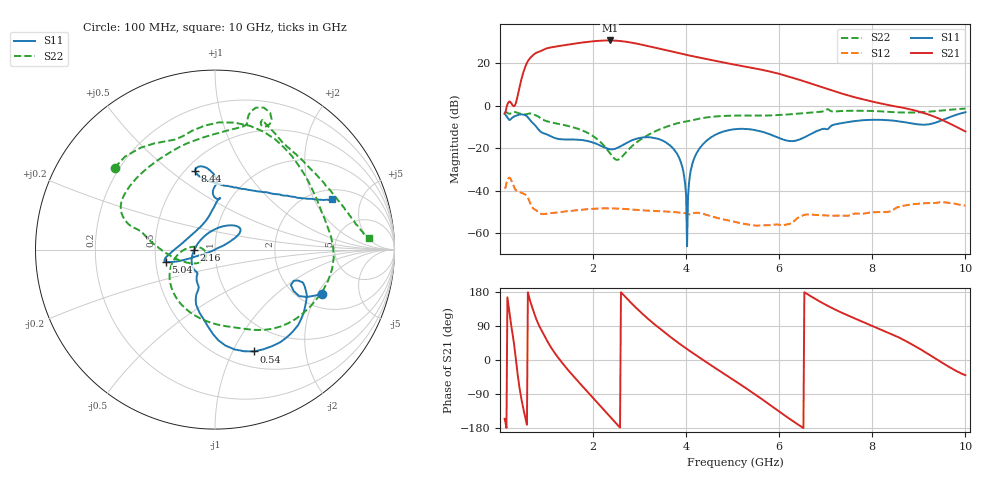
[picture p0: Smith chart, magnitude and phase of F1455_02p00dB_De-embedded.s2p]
! Integrated Device Technology
! Corporate Headquarters
! 6024 Silver Creek Valley Road
! San Jose, CA 95138  USA
! Phone:  1-408-284-8200
! Toll Free:  1-800-223-1366
! Webpage:  http://www.idt.com/
! Timing and RF Division
! 515 Groton Road, Suite 102
! Westford, MA 01886-6024
! Device:  F1455
! Description: 6-bit 0.5 dB Transmit Variable Gain Amplifier
! Frequency:  1400.0 -  2300.00 MHz
! Package:  6x6 mm Thin QFN Plastic Package: 28 pin
! State:  4
! Atten State:  2.0 dB
! Voltage:  +5.00 Volts
! Current:  214.739 mA
! Data:  The device was measured on a the F1455 evaluation board which has
!  individual transmission lines to the RF pins.  Data was collected
!  using a calibrated network analyzer.  The evaluation board was
!  de-embedded using a TRL calibration technique.
!  The reference plane is the edge of the package pin.
!  Pin  1 = CSb
!  Pin  2 = DATA
!  Pin  3 = CLK
!  Pin  4 = RSET
!  Pin  5 = GND
!  Pin  6 = RFIN  = Port 1
!  Pin  7 = GND
!  Pin  8 = NC
!  Pin  9 = NC
!  Pin 10 = NC
!  Pin 11 = NC
!  Pin 12 = NC
!  Pin 13 = NC
!  Pin 14 = /STBY
!  Pin 15 = GND
!  Pin 16 = RFOUT  = Port 2
!  Pin 17 = GND
!  Pin 18 = NC
!  Pin 19 = NC
!  Pin 20 = NC
!  Pin 21 = GND
!  Pin 22 = NC
!  Pin 23 = GND
!  Pin 24 = NC
!  Pin 25 = NC
!  Pin 26 = NC
!  Pin 27 = GND
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# GHz S dB R 50
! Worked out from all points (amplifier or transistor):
!   496 points, 100 MHz to 10 GHz, reference 50 ohm
!   highest |S21| = 30.8 dB at 2.36 GHz (marker M1)
!   |S21| within 3 dB of that: 1.169 GHz to 3.251 GHz (2.082 GHz wide, 94.2 % of centre)
!   unconditionally stable (mu >= 1): start of sweep to end of sweep
!   at 1.74 GHz: K = 4.15, MAG = 30.2 dB, |S12| = -48.9 dB
!   at 5.06 GHz: K = 17.75, MAG = 21.6 dB, |S12| = -54.8 dB
!   at 10 GHz: K = 56.40, MAG = -3.0 dB, |S12| = -47.0 dB
!   S11 on the Smith chart (normalised r, x): 100 MHz: 2.58, -2.20; 540 MHz: 0.68, -1.22; 2.16 GHz: 0.79, -0.00; 5.04 GHz: 0.57, -0.08; 8.44 GHz: 0.56, +0.61; 10 GHz: 2.49, +2.80
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0.1  -3.81 -22.8  -3.44 -155.2  -38.93 40.0  -2.83 140.8
0.4  -4.20 -38.8  6.84 -56.6  -40.45 -111.8  -3.42 50.4
0.54  -4.32 -68.9  18.17 -149.4  -41.75 -157.8  -4.02 19.8
0.7  -7.98 -98.5  23.68 135.9  -48.00 154.2  -3.83 -20.5
0.96  -13.09 -114.6  26.73 62.9  -50.95 124.9  -6.86 -73.8
1.14  -14.80 -124.1  27.72 25.1  -50.44 102.2  -7.96 -97.4
1.34  -15.75 -127.5  28.47 -8.0  -49.93 80.7  -8.86 -120.4
1.76  -16.06 -143.3  29.82 -67.6  -48.89 46.0  -11.46 -157.8
1.96  -17.00 -156.9  30.34 -94.4  -48.54 32.2  -13.65 -172.7
2.16  -18.77 -179.2  30.71 -121.5  -48.29 19.3  -17.03 174.9
2.36  -20.42 142.7  30.83 -148.8  -48.28 6.7  -22.20 173.5
2.6  -18.93 90.4  30.52 178.8  -48.47 -7.0  -24.43 -144.0
2.9  -15.70 55.5  29.50 140.7  -48.93 -21.2  -17.79 -143.6
3.4  -15.52 34.1  27.09 86.2  -49.60 -40.4  -11.36 -175.5
4.04  -43.24 -152.8  23.88 27.1  -51.06 -64.4  -7.18 165.8
5.04  -11.00 -166.0  19.45 -54.4  -54.58 -99.4  -4.57 149.0
5.06  -10.94 -166.3  19.37 -56.0  -54.77 -99.7  -4.57 148.4
5.9  -14.27 171.8  15.67 -127.1  -55.96 -101.9  -4.41 111.0
6.7  -12.99 93.3  10.40 166.6  -51.23 -132.2  -3.13 78.2
8.36  -6.78 103.8  0.31 71.1  -49.83 174.1  -2.79 62.2
8.44  -6.92 104.2  -0.03 67.1  -49.08 176.1  -2.91 59.9
10  -2.99 23.3  -12.04 -40.3  -46.99 87.8  -1.28 4.5
